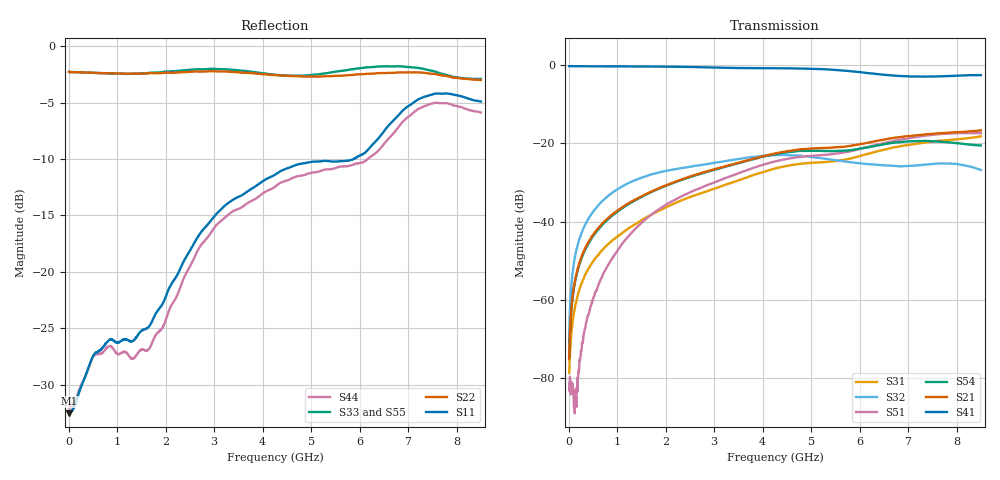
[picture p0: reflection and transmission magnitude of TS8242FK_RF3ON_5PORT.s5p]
! Created with skrf (http://scikit-rf.org).
# Hz S RI R 50.0
!freq ReS11 ImS11 ReS12 ImS12 ReS13 ImS13
! ReS14 ImS14 ReS15 ImS15
! ReS21 ImS21 ReS22 ImS22 ReS23 ImS23
! ReS24 ImS24 ReS25 ImS25
! ReS31 ImS31 ReS32 ImS32 ReS33 ImS33
! ReS34 ImS34 ReS35 ImS35
! ReS41 ImS41 ReS42 ImS42 ReS43 ImS43
! ReS44 ImS44 ReS45 ImS45
! ReS51 ImS51 ReS52 ImS52 ReS53 ImS53
! ReS54 ImS54 ReS55 ImS55
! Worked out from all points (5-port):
!   1601 points, 10 MHz to 8.5 GHz, reference 50 ohm
!   strongest paths, dB at 10 MHz, 2.132 GHz, 4.255 GHz, 6.378 GHz, 8.5 GHz:
!     S41: -0.3, -0.4, -0.8, -2.3, -2.5
!     S21: -75.2, -30.1, -22.6, -19.3, -16.7
!     S54: -74.7, -30.2, -22.8, -20.5, -20.5
!     S51: -83.1, -34.8, -24.6, -20.3, -17.4
!     S32: -71.1, -26.7, -23.1, -25.5, -26.8
!     S31: -78.6, -35.6, -26.4, -22.0, -18.2
!   lowest |S11| = -32.5 dB at 15.31 MHz (marker M1), VSWR 1.05, Z = 52.4 - j0.119 ohm
!   |S11| at or under -10 dB: start of sweep to 5.873 GHz
